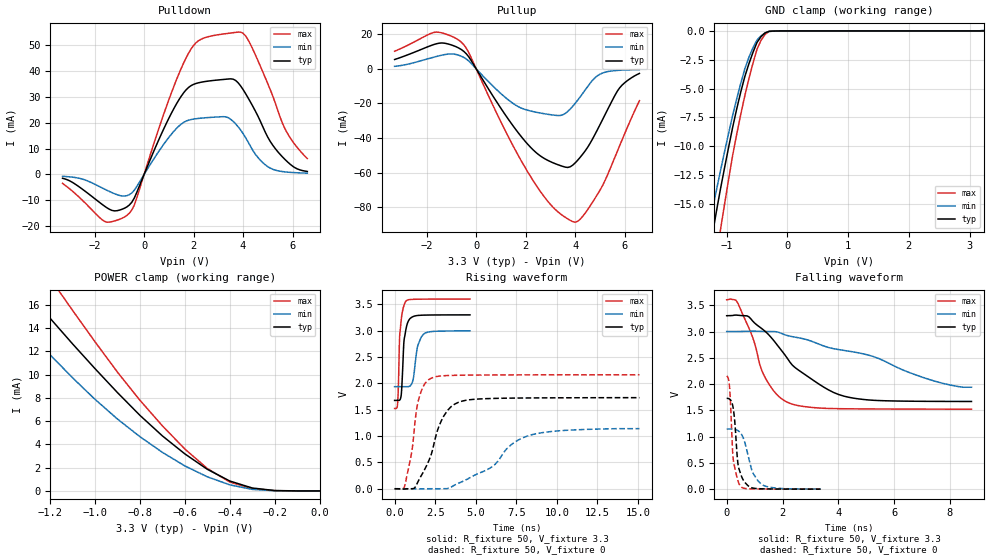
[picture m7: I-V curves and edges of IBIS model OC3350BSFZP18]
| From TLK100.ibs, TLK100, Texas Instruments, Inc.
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|   Model Cell OC3350BSFZP18
[Model]   OC3350BSFZP18
Model_type   I/O
Polarity   Non-Inverting
Enable   Active-Low
Vinl =  0.8V
Vinh =  2V
Cref =  15.0000pF
Rref =  100
Vref =  0V
Vmeas =  1.65
C_comp   1.572001p   1.534781p   1.612244p
[Model Spec]
Vinl   0.8V   0.8V   0.8V
Vinh   2V   2V   2V
[Temperature Range]   25   125   -40
[Voltage Range]   3.3   3   3.6
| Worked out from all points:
|   slope of the pulldown table from 0 to 0.495 V, typ, clamps not added: 44 ohm
|   slope of the pullup table from 0 to 0.495 V, typ, clamps not added: 42.8 ohm
|   GND clamp passes 1 mA (typ) near -0.50 V on its own axis
|   POWER clamp passes 1 mA (typ) near -0.41 V on its own axis
|   rising waveform, R_fixture 50, V_fixture 3.3: 20-80 % time 214ps typ, 335ps min, 169ps max; typ from 1.68 V to 3.3 V
|   rising waveform, R_fixture 50, V_fixture 0: 20-80 % time 1.22ns typ, 2.8ns min, 625ps max; typ from 0 V to 1.73 V
|   falling waveform, R_fixture 50, V_fixture 3.3: 20-80 % time 1.88ns typ, 3.72ns min, 897ps max; typ from 3.3 V to 1.67 V
|   falling waveform, R_fixture 50, V_fixture 0: 20-80 % time 194ps typ, 398ps min, 154ps max; typ from 1.73 V to 0.001 V
[POWER_clamp]
|   voltage   I(typ)   I(min)   I(max)
-3.3V     74.53mA    56.62mA    89.71mA
-1.433V   20.46mA    16.56mA    24.82mA
-1.3V     17.11mA    13.73mA    21.04mA
-1.267V   16.35mA    13.05mA    20.11mA
-1.167V   14.08mA    11.02mA    17.33mA
-1.133V   13.35mA    10.37mA    16.41mA
-800mV    6.485mA    4.653mA    7.778mA
-600mV    3.177mA    2.145mA    3.594mA
-500mV    1.856mA    1.21mA     1.925mA
-400mV    849.6uA    521.8uA    759.7uA
-300mV    251.9uA    131.3uA    193.7uA
0V        16.41nA    105nA      16.59nA
[Pulldown]
|   voltage   I(typ)   I(min)   I(max)
-3.3V     -1.51mA    -734.9uA   -3.488mA
-1.6V     -12.28mA   -5.696mA   -18.17mA
-700mV    -12.58mA   -8.234mA   -15.87mA
-400mV    -9.19mA    -6.127mA   -11.9mA
1.2V      25.39mA    16.63mA    33.95mA
1.9V      34.3mA     21.2mA     48.49mA
3.3V      36.76mA    22.24mA    54.37mA
3.8V      35.41mA    18.42mA    54.98mA
4.2V      29.63mA    12.59mA    52.05mA
5V        14.38mA    2.993mA    35.05mA
5.7V      5.726mA    960.8uA    17.55mA
6.6V      1.128mA    471.3uA    6.106mA
[Pullup]
|   voltage   I(typ)   I(min)   I(max)
-3.3V     5.393mA    1.437mA    10.17mA
-1.7V     14.11mA    6.797mA    21.07mA
-600mV    11.14mA    7.287mA    15.39mA
-300mV    6.902mA    4.521mA    9.337mA
1.3V      -29.12mA   -17.95mA   -39.24mA
2.3V      -46.77mA   -24.67mA   -64.54mA
3.4V      -55.87mA   -26.94mA   -83.73mA
4V        -54.36mA   -19.96mA   -88.58mA
4.4V      -47.51mA   -12.35mA   -83.49mA
5V        -32.4mA    -3.137mA   -70.19mA
5.8V      -10.97mA   -830.7uA   -44.42mA
6.6V      -2.645mA   -449.1uA   -18.4mA
[GND_clamp]
|   voltage   I(typ)   I(min)   I(max)
-3.3V     -90.23mA   -69.53mA   -106.7mA
-1.3V     -19.77mA   -17.24mA   -24mA
-1.233V   -17.66mA   -15.52mA   -21.73mA
-1.167V   -15.64mA   -13.81mA   -19.48mA
-1.1V     -13.7mA    -12.12mA   -17.24mA
-1.033V   -11.88mA   -10.48mA   -15.04mA
-900mV    -8.367mA   -7.325mA   -10.8mA
-700mV    -3.963mA   -3.292mA   -5.626mA
-500mV    -1.004mA   -793.6uA   -1.596mA
-366.7mV  -172.3uA   -169.6uA   -300.4uA
-166.7mV  -4.07uA    -5.719uA   -4.513uA
3.233V    -14.17nA   54.69uA    -20.75nA
[Ramp]
| variable   typ   min   max
dV/dt_f  0.9872792/1.894677n   0.6915556/4.043168n   1.258921/0.9046261n
dV/dt_r   1.041916/1.225344n   0.7009482/2.893656n   1.302382/0.6268036n
R_load = 50
[Rising Waveform]
R_fixture = 50
V_fixture = 3.3
V_fixture_min = 3
V_fixture_max = 3.6
|   time   V(typ)   V(min)   V(max)
0s        1.676V     1.937V     1.523V
180ps     1.676V     1.937V     1.594V
312ps     1.682V     1.937V     2.903V
396ps     1.754V     1.937V     3.171V
570ps     2.772V     1.937V     3.472V
660ps     2.956V     1.937V     3.542V
1.086ns   3.26V      2.014V     3.594V
1.428ns   3.288V     2.717V     3.597V
1.77ns    3.295V     2.93V      3.598V
4.644ns   3.3V       2.997V     3.6V
[Rising Waveform]
R_fixture = 50
V_fixture = 0
V_fixture_min = 0
V_fixture_max = 0
|   time   V(typ)   V(min)   V(max)
0s        18.51uV    15.96uV    -2.058uV
624ps     -4.876mV   18.7uV     55.37mV
1.062ns   412uV      -705.3uV   713.4mV
1.44ns    132.8mV    -3.947mV   1.644V
1.806ns   338.8mV    -780.9uV   1.964V
2.262ns   656.2mV    23.75uV    2.098V
3.024ns   1.377V     423.1uV    2.145V
4.152ns   1.662V     132.9mV    2.155V
8.178ns   1.723V     1.001V     2.161V
15.08ns   1.728V     1.141V     2.162V
[Falling Waveform]
R_fixture = 50
V_fixture = 3.3
V_fixture_min = 3
V_fixture_max = 3.6
|   time   V(typ)   V(min)   V(max)
0s        3.301V     3V         3.604V
396ps     3.311V     3.001V     3.545V
924ps     3.205V     3.007V     2.901V
1.32ns    3.03V      3.002V     2.184V
1.752ns   2.784V     2.998V     1.827V
2.178ns   2.487V     2.924V     1.653V
3.468ns   1.945V     2.727V     1.54V
4.368ns   1.749V     2.627V     1.53V
7.44ns    1.671V     2.058V     1.523V
8.772ns   1.669V     1.94V      1.522V
[Falling Waveform]
R_fixture = 50
V_fixture = 0
V_fixture_min = 0
V_fixture_max = 0
|   time   V(typ)   V(min)   V(max)
0s        1.729V     1.144V     2.154V
102ps     1.715V     1.145V     1.948V
204ps     1.619V     1.144V     810.3mV
240ps     1.521V     1.142V     544.9mV
396ps     516.9mV    1.116V     176mV
492ps     304.1mV    1.073V     58.52mV
630ps     144.8mV    922.2mV    16.14mV
912ps     24.84mV    346.2mV    5.558mV
1.224ns   7.732mV    103.2mV    2.954mV
3.366ns   884.4uV    3.029mV    228uV
